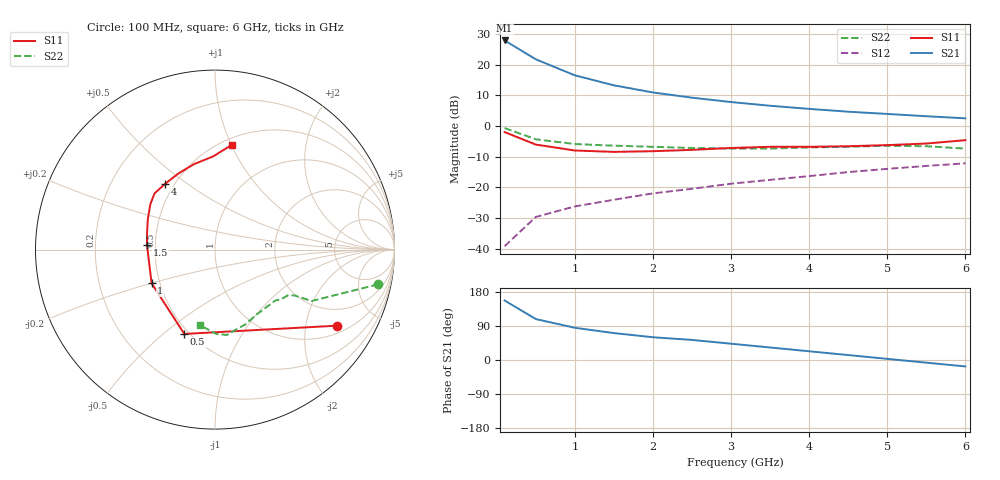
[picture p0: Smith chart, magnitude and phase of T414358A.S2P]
!AT-41435
!S AND NOISE PARAMETERS at Vce=8V  Ic=10mA.  LAST UPDATED 07-21-92
# ghz s ma r 50
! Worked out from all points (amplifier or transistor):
!   13 points, 100 MHz to 6 GHz, reference 50 ohm
!   highest |S21| = 28.0 dB at 100 MHz (marker M1)
!   |S21| within 3 dB of that: start of sweep to 294.9 MHz
!   unconditionally stable (mu >= 1): 1.189 GHz to 4.173 GHz
!   at 1 GHz: K = 0.94, MSG = 21.4 dB, |S12| = -26.2 dB
!   at 3 GHz: K = 1.11, MAG = 11.3 dB, |S12| = -18.8 dB
!   at 6 GHz: K = 0.77, MSG = 7.3 dB, |S12| = -12.1 dB
!   lowest NFmin = 1.20 dB at 100 MHz
!   S11 on the Smith chart (normalised r, x): 100 MHz: 1.27, -2.99; 500 MHz: 0.47, -0.59; 1 GHz: 0.45, -0.20; 1.5 GHz: 0.45, +0.03; 4 GHz: 0.45, +0.42; 6 GHz: 0.56, +1.00
0.1  0.8 -32.0  24.99 157.0  0.011 82.0  0.93 -12.0
0.5  0.5 -110.0  12.3 108.0  0.033 52.0  0.61 -28.0
1  0.4 -152.0  6.73 85.0  0.049 56.0  0.51 -30.0
1.5  0.38 176.0  4.63 71.0  0.063 59.0  0.48 -32.0
2  0.39 166.0  3.54 60.0  0.08 58.0  0.46 -37.0
2.5  0.41 156.0  2.91 53.0  0.095 61.0  0.44 -40.0
3  0.44 145.0  2.47 43.0  0.115 61.0  0.43 -48.0
3.5  0.46 137.0  2.15 33.0  0.133 58.0  0.43 -58.0
4  0.46 127.0  1.91 23.0  0.153 53.0  0.45 -68.0
4.5  0.47 116.0  1.72 13.0  0.178 50.0  0.46 -75.0
5  0.49 104.0  1.58 3.0  0.201 47.0  0.48 -82.0
5.5  0.52 91.0  1.45 -7.0  0.224 40.0  0.47 -89.0
6  0.59 81.0  1.34 -17.0  0.247 36.0  0.43 -101.0
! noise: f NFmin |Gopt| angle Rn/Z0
0.1  1.2  0.12  3  0.17
0.5  1.2  0.1  14  0.17
1  1.3  0.05  28  0.17
2  1.7  0.3  -154  0.16
4  3  0.54  -118  0.35
